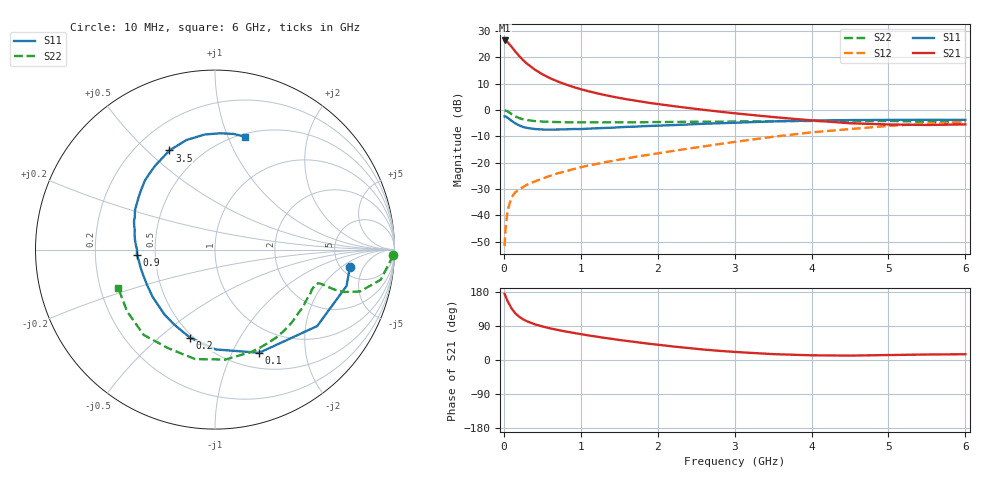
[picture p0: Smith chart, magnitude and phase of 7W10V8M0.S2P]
! Infineon Technologies  Discrete & RF Semiconductors
! BFS17W
! Si NPN RF Bipolar Junction Transistor in SOT323
! VCE = 10 V  IC = 8 mA
! Common Emitter S-Parameters:  August  1999
# GHz  S  MA  R  50
!  f  S11  S21  S12  S22
! GHz  MAG  ANG  MAG  ANG  MAG  ANG  MAG  ANG
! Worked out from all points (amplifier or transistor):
!   36 points, 10 MHz to 6 GHz, reference 50 ohm
!   highest |S21| = 26.4 dB at 10 MHz (marker M1)
!   |S21| within 3 dB of that: start of sweep to 116.6 MHz
!   unconditionally stable (mu >= 1): 485.3 MHz to 2.18 GHz; 5.511 GHz to end of sweep
!   at 250 MHz: K = 0.71, MSG = 24.1 dB, |S12| = -29.3 dB
!   at 1.4 GHz: K = 1.17, MAG = 9.8 dB, |S12| = -19.4 dB
!   at 6 GHz: K = 1.03, MAG = -1.6 dB, |S12| = -4.5 dB
!   S11 on the Smith chart (normalised r, x): 10 MHz: 5.94, -2.75; 100 MHz: 0.68, -1.28; 200 MHz: 0.48, -0.64; 900 MHz: 0.39, -0.03; 3.5 GHz: 0.34, +0.59; 6 GHz: 0.53, +1.15
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0.01  0.7574 -7.5  20.92 174.8  0.0026 80.3  0.9933 -1.8
0.02  0.7605 -15.4  20.8 169.3  0.0053 84.8  0.9741 -4.4
0.05  0.7112 -36.8  19.28 154.9  0.0125 75.2  0.9386 -10.3
0.1  0.6254 -66.8  15.9 136.2  0.022 62.8  0.8408 -16.1
0.15  0.5562 -89.6  12.85 122.9  0.0274 55.7  0.7562 -18.2
0.2  0.5103 -105.8  10.58 114.1  0.0311 55.8  0.7034 -18.5
0.25  0.476 -118.3  8.862 107.4  0.0343 54.2  0.6668 -18.3
0.3  0.4581 -128.1  7.601 102.3  0.0381 55.0  0.6457 -18.1
0.4  0.4362 -142.8  5.888 94.4  0.0438 57.1  0.6166 -17.9
0.5  0.4265 -152.8  4.784 88.6  0.0499 59.1  0.6041 -18.1
0.6  0.4247 -160.4  4.021 83.6  0.056 61.2  0.5958 -18.8
0.7  0.4266 -166.5  3.485 79.3  0.0628 63.0  0.5901 -19.9
0.9  0.4362 -176.1  2.743 71.8  0.075 65.3  0.5837 -22.7
1.1  0.4434 175.8  2.273 64.8  0.0888 66.8  0.5828 -26.1
1.3  0.4561 169.1  1.943 58.7  0.1017 68.1  0.5817 -30.1
1.6  0.4789 160.4  1.597 50.3  0.1207 69.9  0.5836 -36.2
2.2  0.5171 145.2  1.188 35.7  0.1671 72.7  0.5938 -50.1
2.8  0.5601 130.4  0.933 24.2  0.2253 72.8  0.6014 -65.5
3.5  0.6079 114.7  0.736 15.5  0.3104 69.1  0.6157 -84.6
4.5  0.6438 95.1  0.56 11.6  0.4347 57.6  0.6082 -115.4
5.5  0.6529 80.7  0.52 14.5  0.5498 44.2  0.5987 -144.9
6  0.6502 75.1  0.533 15.2  0.5953 37.6  0.5802 -158.2
